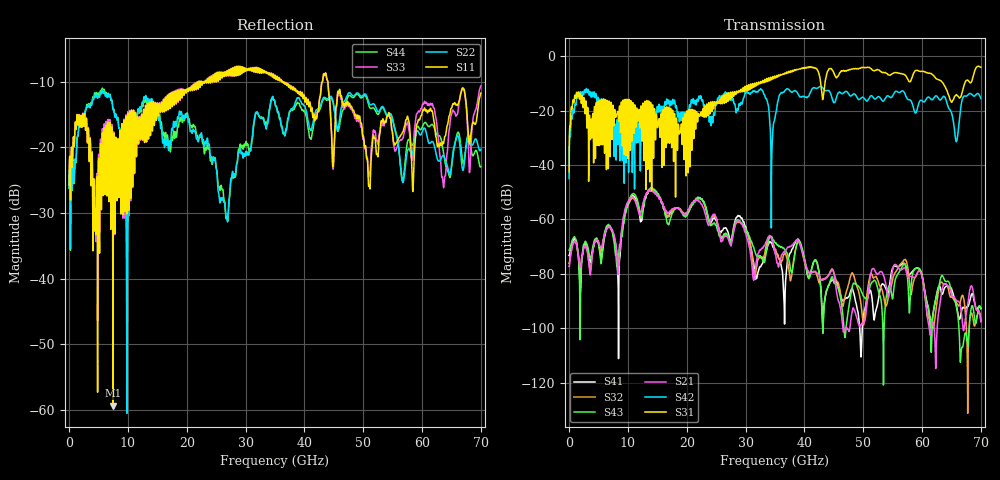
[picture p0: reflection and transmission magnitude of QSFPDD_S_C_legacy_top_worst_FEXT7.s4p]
! AWR Design Environment (8415) Fri Dec 21 09:39:33 2018
! Document = 'CHANNEL TEST'
! nPorts: 4, nXvals: 7001
# HZ S DB R 50
!Freq DBS11 AngS11 DBS12 AngS12 DBS13 AngS13 DBS14 AngS14
!	DBS21 AngS21 DBS22 AngS22 DBS23 AngS23 DBS24 AngS24
!	DBS31 AngS31 DBS32 AngS32 DBS33 AngS33 DBS34 AngS34
!	DBS41 AngS41 DBS42 AngS42 DBS43 AngS43 DBS44 AngS44
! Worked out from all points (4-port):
!   7000 points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, 10 MHz to 70 GHz, reference 50 ohm
!   strongest paths, dB at 10 MHz, 17.51 GHz, 35.01 GHz, 52.51 GHz, 70 GHz:
!     S31: -42.4, -23.4, -7.5, -5.0, -4.0
!     S42: -45.0, -17.1, -22.4, -14.9, -15.5
!     S21: -77.3, -56.2, -72.6, -80.1, -97.6
!     S43: -71.3, -57.9, -68.6, -85.8, -92.9
!     S32: -76.1, -57.0, -71.0, -82.5, -97.3
!     S41: -73.2, -56.3, -71.8, -90.3, -92.6
!   lowest |S11| = -59.3 dB at 7.44 GHz (marker M1), VSWR 1.00, Z = 50.1 - j0.0606 ohm
!   |S11| at or under -10 dB: start of sweep to 22.09 GHz; 36.3 GHz to 43.07 GHz (6.77 GHz wide, 17.1 % of centre); 43.97 GHz to end of sweep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
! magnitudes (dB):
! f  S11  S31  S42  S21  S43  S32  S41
! 10 MHz  -25.8  -42.4  -45.0  -77.3  -71.3  -76.1  -73.2
! 1.69 GHz  -15.0  -14.3  -13.4  -75.5  -77.3  -76.6  -77.0
! 7.44 GHz  -59.3  -18.1  -22.4  -64.5  -65.8  -65.4  -64.8
! 9.77 GHz  -22.5  -19.1  -34.3  -54.5  -55.9  -56.2  -55.1
! 13.01 GHz  -13.6  -22.8  -23.2  -51.4  -52.0  -51.7  -52.3
! 31.4 GHz  -8.5  -11.4  -13.0  -82.3  -70.5  -79.1  -76.3
! 70 GHz  -11.8  -4.0  -15.5  -97.6  -92.9  -97.3  -92.6
